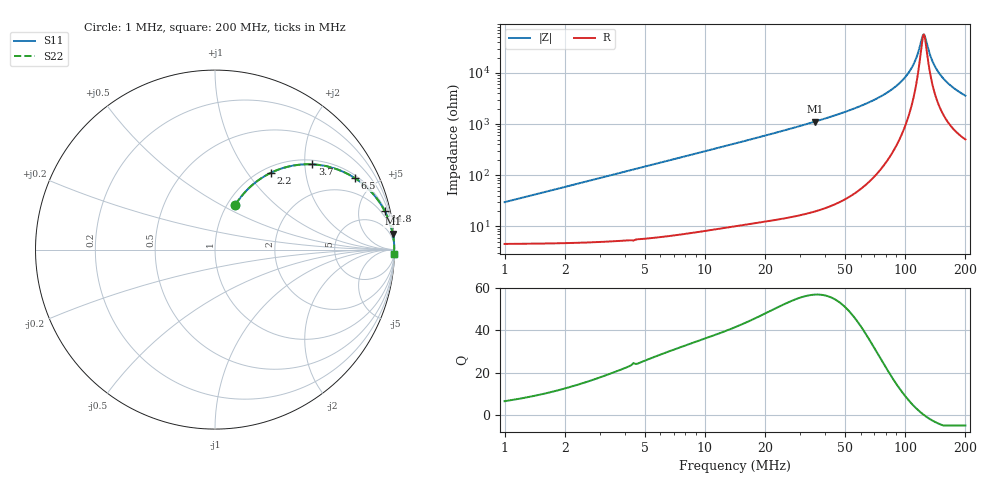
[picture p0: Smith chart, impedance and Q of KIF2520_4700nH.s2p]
!version-2
!date-12.2020
!Series
# MHz S RI R 50
!Freq ReS11 ImS11 ReS21 ImS21 ReS12 ImS12 ReS22 ImS22
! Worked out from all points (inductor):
!   1991 points, 1 MHz to 200 MHz, reference 50 ohm
!   read as one part in series: L = 4.69 uH near 1.9 MHz
!   highest Q = 56.9 at 35.5 MHz (marker M1), where L = 5.01 uH
!   self-resonance near 124 MHz
!   S11 on the Smith chart (normalised r, x): 1 MHz: 1.09, +0.59; 2.2 MHz: 1.10, +1.30; 3.7 MHz: 1.10, +2.18; 6.5 MHz: 1.13, +3.83; 14.8 MHz: 1.21, +8.75; 200 MHz: 11, -71
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1  0.1142 0.25  0.8858 -0.25  0.8858 -0.25  0.1142 0.25
2.2  0.3102 0.4273  0.6898 -0.4273  0.6898 -0.4273  0.3102 0.4273
3.7  0.542 0.4749  0.458 -0.4749  0.458 -0.4749  0.542 0.4749
5  0.6786 0.4479  0.3214 -0.4479  0.3214 -0.4479  0.6786 0.4479
6.5  0.7782 0.399  0.2218 -0.399  0.2218 -0.399  0.7782 0.399
9.8  0.8862 0.3039  0.1138 -0.3039  0.1138 -0.3039  0.8862 0.3039
14.8  0.9458 0.2149  0.0542 -0.2149  0.0542 -0.2149  0.9458 0.2149
23.1  0.977 0.1403  0.023 -0.1403  0.023 -0.1403  0.977 0.1403
34.2  0.9898 0.0922  0.0102 -0.0922  0.0102 -0.0922  0.9898 0.0922
35.5  0.9905 0.0884  0.00945 -0.0884  0.00945 -0.0884  0.9905 0.0884
67.4  0.9976 0.0361  0.00235 -0.0361  0.00235 -0.0361  0.9976 0.0361
87  0.9984 0.0201  0.00159 -0.0201  0.00159 -0.0201  0.9984 0.0201
100.5  0.9985 0.0118  0.0015 -0.0118  0.0015 -0.0118  0.9985 0.0118
112.2  0.9984 0.00557  0.00158 -0.00557  0.00158 -0.00557  0.9984 0.00557
121.7  0.9983 0.00104  0.00173 -0.00104  0.00173 -0.00104  0.9983 0.00104
123.4  0.9982 0.000271  0.00176 -0.000271  0.00176 -0.000271  0.9982 0.000271
125.7  0.9982 -0.000754  0.00181 0.000754  0.00181 0.000754  0.9982 -0.000754
133.7  0.998 -0.00418  0.002 0.00418  0.002 0.00418  0.998 -0.00418
139.5  0.9978 -0.00654  0.00215 0.00654  0.00215 0.00654  0.9978 -0.00654
146.8  0.9976 -0.00939  0.00238 0.00939  0.00238 0.00939  0.9976 -0.00939
166.9  0.9969 -0.0167  0.0031 0.0167  0.0031 0.0167  0.9969 -0.0167
200  0.9954 -0.0273  0.00461 0.0273  0.00461 0.0273  0.9954 -0.0273
